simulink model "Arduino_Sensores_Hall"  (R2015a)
settings: Solver=ode45  StartTime=0.0  StopTime=10.0  RelTol=1e-3
libraries: arduinolib x10, dspsigops x9, simulink x7

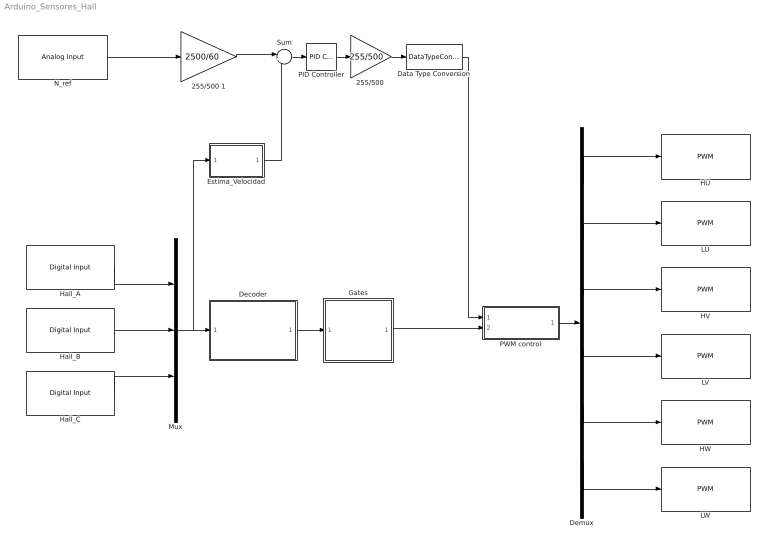
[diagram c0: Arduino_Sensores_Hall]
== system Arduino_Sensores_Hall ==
  "255/500 " : Gain  Gain=255/500
  255/500 1 : Gain  Gain=2500/60
  Data Type Conversion : DataTypeConversion  OutDataTypeStr=int16  RndMeth=Round
  Decoder : Subsystem
  Demux : Demux  Outputs=6
  Estima_Velocidad : Subsystem
  Gates : Subsystem
  HU : arduinolib/PWM  pinNumber=3  blockPlatform=arduino
  HV : arduinolib/PWM  pinNumber=6  blockPlatform=arduino
  HW : arduinolib/PWM  pinNumber=10  blockPlatform=arduino
  Hall_A : arduinolib/Digital Input  pinNumber=8  sampleTime=1  blockPlatform=arduino
  Hall_B : arduinolib/Digital Input  pinNumber=12  sampleTime=1  blockPlatform=arduino
  Hall_C : arduinolib/Digital Input  pinNumber=13  sampleTime=1  blockPlatform=arduino
  LU : arduinolib/PWM  pinNumber=5  blockPlatform=arduino
  LV : arduinolib/PWM  pinNumber=9  blockPlatform=arduino
  LW : arduinolib/PWM  pinNumber=11  blockPlatform=arduino
  Mux : Mux  Inputs=3
  N_ref : arduinolib/Analog Input  pinNumber=0  sampleTime=1  blockPlatform=arduino
  PID Controller : simulink/Continuous/PID Controller  Controller=PID  TimeDomain=Continuous-time  SampleTime=-1  IntegratorMethod=Forward Euler  FilterMethod=Forward Euler  Form=Parallel  UseFilter=on  ControllerParametersSource=internal  P=500  I=0.1  D=0.08  N=1  InitialConditionSource=internal  InitialConditionForIntegrator=0  InitialConditionForFilter=0  ExternalReset=none  LimitOutput=off  UpperSaturationLimit=inf  LowerSaturationLimit=-inf  LinearizeAsGain=on  AntiWindupMode=none  Kb=1  TrackingMode=off  Kt=1  PParamMin=[]  PParamMax=[]  IParamMin=[]  IParamMax=[]  DParamMin=[]  DParamMax=[]  NParamMin=[]  NParamMax=[]  KbParamMin=[]  KbParamMax=[]  KtParamMin=[]  KtParamMax=[]  POutMin=[]  POutMax=[]  IOutMin=[]  IOutMax=[]  DOutMin=[]  DOutMax=[]  NOutMin=[]  NOutMax=[]  KbOutMin=[]  KbOutMax=[]  KtOutMin=[]  KtOutMax=[]  IntegratorOutMin=[]  IntegratorOutMax=[]  FilterOutMin=[]  FilterOutMax=[]  SumOutMin=[]  SumOutMax=[]  SumI1OutMin=[]  SumI1OutMax=[]  SumI2OutMin=[]  SumI2OutMax=[]  SumI3OutMin=[]  SumI3OutMax=[]  SumDOutMin=[]  SumDOutMax=[]  SaturationOutMin=[]  SaturationOutMax=[]  IntegratorContinuousStateAttributes=''  IntegratorStateMustResolveToSignalObject=off  IntegratorRTWStateStorageClass=Auto  FilterContinuousStateAttributes=''  FilterStateMustResolveToSignalObject=off  FilterRTWStateStorageClass=Auto  DifferentiatorICPrevScaledInput=0  DifferentiatorOutMin=[]  DifferentiatorOutMax=[]
  PWM control : Subsystem
  Sum : Sum  Inputs=|+-
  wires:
  Hall_B/1 -> Mux/2
  Hall_A/1 -> Mux/1
  Hall_C/1 -> Mux/3
  Mux/1 -> Estima_Velocidad/1(Hall), Decoder/1("Hall ")
  Gates/1(Gates) -> PWM control/2(Gates)
  Sum/1 -> PID Controller/1
  PID Controller/1 -> "255/500 "/1
  Decoder/1(emf_abc) -> Gates/1("emf_abc ")
  "255/500 "/1 -> Data Type Conversion/1
  Data Type Conversion/1 -> PWM control/1(V control)
  PWM control/1(Pulsos) -> Demux/1
  Demux/1 -> HU/1
  Demux/2 -> LU/1
  Demux/3 -> HV/1
  Demux/4 -> LV/1
  Demux/5 -> HW/1
  Demux/6 -> LW/1
  Estima_Velocidad/1(N_est) -> Sum/2
  255/500 1/1 -> Sum/1
  N_ref/1 -> 255/500 1/1

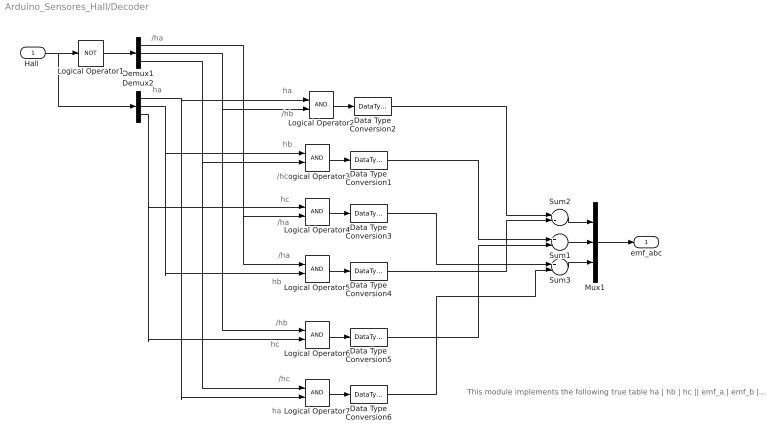
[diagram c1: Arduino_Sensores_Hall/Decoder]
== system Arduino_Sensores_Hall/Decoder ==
  note: /ha
  note: ha
  note: ha
  note: /hb
  note: hb
  note: /hc
  note: hc
  note: /ha
  note: /ha
  note: hb
  note: /hb
  note: hc
  note: /hc
  note: ha
  note: This module implements the following true table ha | hb | hc || emf_a | emf_b | emf_c -------------------------------------------------------------------------------- 0 0 0 0 0 0 0 0 1 0 -1 +1 0 1 0 -1 +1 0 0 1 1 -1 0 +1 1 0 0 +1 0 -1 1 0 1 +1 -1 0 1 1 0 0 +1 -1 1 1 1 0 0 0
  "Hall " : Inport
  Data Type Conversion{1..6} (6 alike) : DataTypeConversion
  Demux1 : Demux  Outputs=3
  Demux2 : Demux  Outputs=3
  Logical Operator1 : Logic  Operator=NOT  AllPortsSameDT=off  OutDataTypeStr=boolean
  Logical Operator{2..7} (6 alike) : Logic  AllPortsSameDT=off  OutDataTypeStr=boolean
  Mux1 : Mux  Inputs=3
  Sum1 : Sum  Inputs=+-  OutDataTypeStr=double
  Sum2 : Sum  Inputs=+-  OutDataTypeStr=double
  Sum3 : Sum  Inputs=+-  OutDataTypeStr=double
  emf_abc : Outport
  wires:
  "Hall "/1 -> Logical Operator1/1, Demux2/1
  Logical Operator1/1 -> Demux1/1
  Demux2/3 -> Logical Operator4/1, Logical Operator6/2
  Demux2/2 -> Logical Operator3/1, Logical Operator5/2
  Demux2/1 -> Logical Operator2/1, Logical Operator7/2
  Demux1/3 -> Logical Operator3/2, Logical Operator7/1
  Demux1/2 -> Logical Operator2/2, Logical Operator6/1
  Demux1/1 -> Logical Operator4/2, Logical Operator5/1
  Logical Operator2/1 -> Data Type Conversion2/1
  Sum2/1 -> Mux1/1
  Sum1/1 -> Mux1/2
  Sum3/1 -> Mux1/3
  Mux1/1 -> emf_abc/1
  Logical Operator3/1 -> Data Type Conversion1/1
  Logical Operator4/1 -> Data Type Conversion3/1
  Logical Operator5/1 -> Data Type Conversion4/1
  Logical Operator6/1 -> Data Type Conversion5/1
  Logical Operator7/1 -> Data Type Conversion6/1
  Data Type Conversion2/1 -> Sum2/1
  Data Type Conversion4/1 -> Sum2/2
  Data Type Conversion1/1 -> Sum1/1
  Data Type Conversion5/1 -> Sum1/2
  Data Type Conversion3/1 -> Sum3/1
  Data Type Conversion6/1 -> Sum3/2

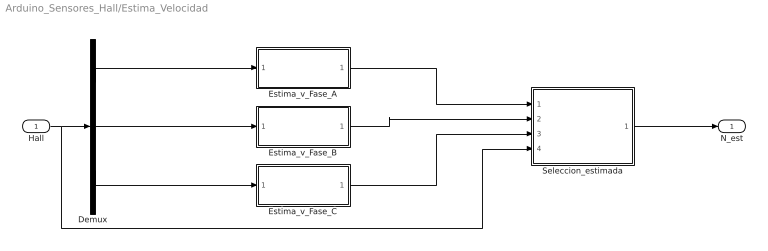
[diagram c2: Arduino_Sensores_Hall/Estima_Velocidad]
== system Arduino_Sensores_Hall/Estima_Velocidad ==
  Hall : Inport
  Demux : Demux  Outputs=3
  Estima_v_Fase_A : Subsystem
  Estima_v_Fase_B : Subsystem
  Estima_v_Fase_C : Subsystem
  Seleccion_estimada : Subsystem
  N_est : Outport
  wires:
  Demux/1 -> Estima_v_Fase_A/1(Hall_i)
  Hall/1 -> Seleccion_estimada/4(Hall), Demux/1
  Demux/3 -> Estima_v_Fase_C/1(Hall_i)
  Demux/2 -> Estima_v_Fase_B/1(Hall_i)
  Estima_v_Fase_A/1(Estimada_i) -> Seleccion_estimada/1(Estimada_A)
  Estima_v_Fase_B/1(Estimada_i) -> Seleccion_estimada/2(Estimada_B)
  Estima_v_Fase_C/1(Estimada_i) -> Seleccion_estimada/3(Estimada_C)
  Seleccion_estimada/1(Out1) -> N_est/1

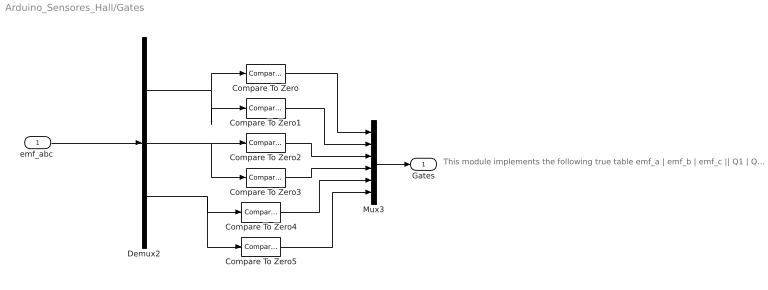
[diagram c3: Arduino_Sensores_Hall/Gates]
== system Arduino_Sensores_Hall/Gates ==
  note: This module implements the following true table emf_a | emf_b | emf_c || Q1 | Q2 | Q3 | Q4 | Q5 | Q6 ------------------------------------------------------------------------------------------------------------------ 0 0 0 0 0 0 0 0 0 0 -1 +1 0 0 0 1 1 0 -1 +1 0 0 1 1 0 0 0 -1 0 +1 0 1 0 0 1 0 +1 0 -1 1 0 0 0 0 1 +1 -1 0 1 0 0 1 0 0 0 +1 -1 0 0 1 0 0 1 0 0 0 0 0 0 0 0 0
  "emf_abc " : Inport
  Compare To Zero : simulink/Logic and Bit Operations/Compare To Zero  relop=>  OutDataTypeStr=boolean  ZeroCross=off
  Compare To Zero1 : simulink/Logic and Bit Operations/Compare To Zero  relop=<  OutDataTypeStr=boolean  ZeroCross=off
  Compare To Zero2 : simulink/Logic and Bit Operations/Compare To Zero  relop=>  OutDataTypeStr=boolean  ZeroCross=off
  Compare To Zero3 : simulink/Logic and Bit Operations/Compare To Zero  relop=<  OutDataTypeStr=boolean  ZeroCross=off
  Compare To Zero4 : simulink/Logic and Bit Operations/Compare To Zero  relop=>  OutDataTypeStr=boolean  ZeroCross=off
  Compare To Zero5 : simulink/Logic and Bit Operations/Compare To Zero  relop=<  OutDataTypeStr=boolean  ZeroCross=off
  Demux2 : Demux  Outputs=3
  Mux3 : Mux  Inputs=6
  Gates : Outport
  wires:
  "emf_abc "/1 -> Demux2/1
  Mux3/1 -> Gates/1
  Demux2/1 -> Compare To Zero/1, Compare To Zero1/1
  Demux2/2 -> Compare To Zero2/1, Compare To Zero3/1
  Demux2/3 -> Compare To Zero4/1, Compare To Zero5/1
  Compare To Zero/1 -> Mux3/1
  Compare To Zero1/1 -> Mux3/2
  Compare To Zero2/1 -> Mux3/3
  Compare To Zero3/1 -> Mux3/4
  Compare To Zero4/1 -> Mux3/5
  Compare To Zero5/1 -> Mux3/6

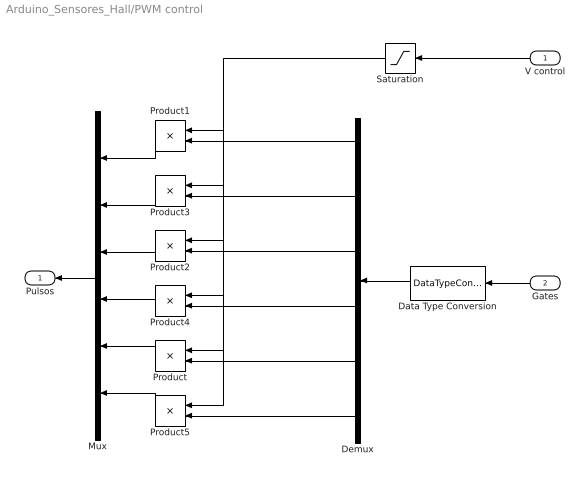
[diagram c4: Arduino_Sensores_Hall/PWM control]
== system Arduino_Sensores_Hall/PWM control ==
  V control : Inport
  Gates : Inport  Port=2
  Data Type Conversion : DataTypeConversion  OutDataTypeStr=double
  Demux : Demux  Outputs=6
  Mux : Mux  Inputs=6
  Product{,1..5} (6 alike) : Product
  Saturation : Saturate  UpperLimit=255  LowerLimit=0
  Pulsos : Outport
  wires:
  Gates/1 -> Data Type Conversion/1
  Data Type Conversion/1 -> Demux/1
  Mux/1 -> Pulsos/1
  Product1/1 -> Mux/1
  Product2/1 -> Mux/3
  Product/1 -> Mux/5
  Demux/5 -> Product/2
  Demux/3 -> Product2/2
  Demux/1 -> Product1/2
  V control/1 -> Saturation/1
  Product5/1 -> Mux/6
  Demux/6 -> Product5/2
  Product4/1 -> Mux/4
  Demux/4 -> Product4/2
  Product3/1 -> Mux/2
  Demux/2 -> Product3/2
  Saturation/1 -> Product3/1, Product4/1, Product/1, Product5/1, Product2/1, Product1/1

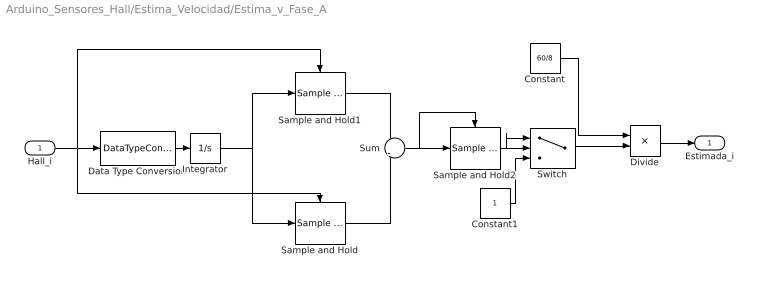
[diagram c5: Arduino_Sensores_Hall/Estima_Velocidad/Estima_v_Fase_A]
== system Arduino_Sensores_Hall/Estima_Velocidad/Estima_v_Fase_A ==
  Hall_i : Inport
  Constant : Constant  Value=60/8
  Constant1 : Constant
  Data Type Conversion : DataTypeConversion  OutDataTypeStr=double
  Divide : Product  Inputs=*/
  Integrator : Integrator
  Sample and Hold : dspsigops/Sample and Hold  trig=Rising edge  initCond=0  latchinput=off
  Sample and Hold1 : dspsigops/Sample and Hold  trig=Falling edge  initCond=0  latchinput=off
  Sample and Hold2 : dspsigops/Sample and Hold  trig=Rising edge  initCond=0  latchinput=off
  Sum : Sum  Inputs=+|-
  Switch : Switch  Criteria=u2 > Threshold
  Estimada_i : Outport
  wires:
  Hall_i/1 -> Data Type Conversion/1, Sample and Hold/Trigger, Sample and Hold1/Trigger
  Integrator/1 -> Sample and Hold1/1, Sample and Hold/1
  Sample and Hold/1 -> Sum/2
  Sample and Hold1/1 -> Sum/1
  Sum/1 -> Sample and Hold2/Trigger, Sample and Hold2/1
  Sample and Hold2/1 -> Switch/1, Switch/2
  Constant/1 -> Divide/1
  Switch/1 -> Divide/2
  Constant1/1 -> Switch/3
  Divide/1 -> Estimada_i/1
  Data Type Conversion/1 -> Integrator/1

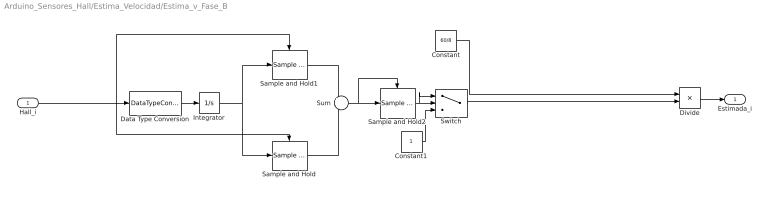
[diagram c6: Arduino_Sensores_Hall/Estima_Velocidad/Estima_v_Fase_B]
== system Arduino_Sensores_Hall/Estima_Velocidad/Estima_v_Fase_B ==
  Hall_i : Inport
  Constant : Constant  Value=60/8
  Constant1 : Constant
  Data Type Conversion : DataTypeConversion  OutDataTypeStr=double
  Divide : Product  Inputs=*/
  Integrator : Integrator
  Sample and Hold : dspsigops/Sample and Hold  trig=Rising edge  initCond=0  latchinput=off
  Sample and Hold1 : dspsigops/Sample and Hold  trig=Falling edge  initCond=0  latchinput=off
  Sample and Hold2 : dspsigops/Sample and Hold  trig=Rising edge  initCond=0  latchinput=off
  Sum : Sum  Inputs=+|-
  Switch : Switch  Criteria=u2 > Threshold
  Estimada_i : Outport
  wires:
  Hall_i/1 -> Sample and Hold/Trigger, Sample and Hold1/Trigger, Data Type Conversion/1
  Integrator/1 -> Sample and Hold1/1, Sample and Hold/1
  Sample and Hold/1 -> Sum/2
  Sample and Hold1/1 -> Sum/1
  Sum/1 -> Sample and Hold2/Trigger, Sample and Hold2/1
  Sample and Hold2/1 -> Switch/1, Switch/2
  Constant/1 -> Divide/1
  Switch/1 -> Divide/2
  Constant1/1 -> Switch/3
  Divide/1 -> Estimada_i/1
  Data Type Conversion/1 -> Integrator/1

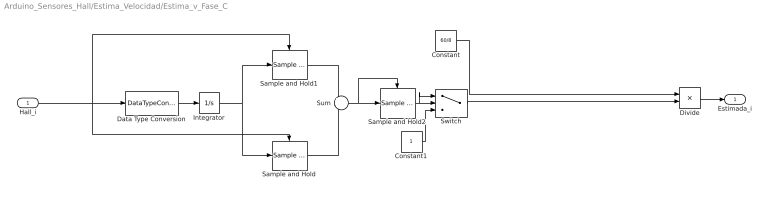
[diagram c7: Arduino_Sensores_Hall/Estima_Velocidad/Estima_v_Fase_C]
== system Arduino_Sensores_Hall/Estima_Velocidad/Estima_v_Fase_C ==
  Hall_i : Inport
  Constant : Constant  Value=60/8
  Constant1 : Constant
  Data Type Conversion : DataTypeConversion  OutDataTypeStr=double
  Divide : Product  Inputs=*/
  Integrator : Integrator
  Sample and Hold : dspsigops/Sample and Hold  trig=Rising edge  initCond=0  latchinput=off
  Sample and Hold1 : dspsigops/Sample and Hold  trig=Falling edge  initCond=0  latchinput=off
  Sample and Hold2 : dspsigops/Sample and Hold  trig=Rising edge  initCond=0  latchinput=off
  Sum : Sum  Inputs=+|-
  Switch : Switch  Criteria=u2 > Threshold  Threshold=3E-5
  Estimada_i : Outport
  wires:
  Hall_i/1 -> Data Type Conversion/1, Sample and Hold/Trigger, Sample and Hold1/Trigger
  Integrator/1 -> Sample and Hold1/1, Sample and Hold/1
  Sample and Hold/1 -> Sum/2
  Sample and Hold1/1 -> Sum/1
  Sum/1 -> Sample and Hold2/Trigger, Sample and Hold2/1
  Sample and Hold2/1 -> Switch/1, Switch/2
  Constant/1 -> Divide/1
  Switch/1 -> Divide/2
  Constant1/1 -> Switch/3
  Divide/1 -> Estimada_i/1
  Data Type Conversion/1 -> Integrator/1

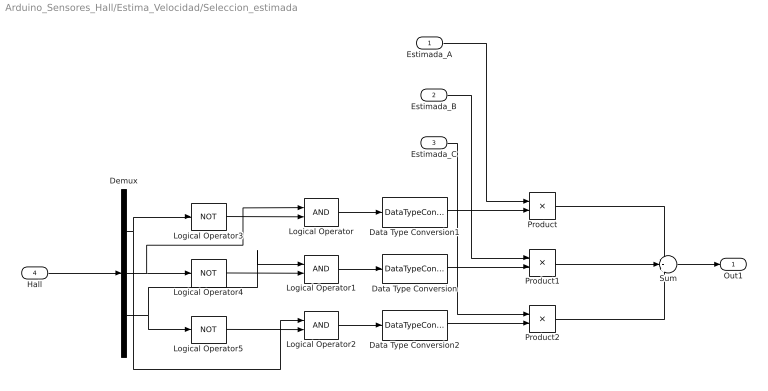
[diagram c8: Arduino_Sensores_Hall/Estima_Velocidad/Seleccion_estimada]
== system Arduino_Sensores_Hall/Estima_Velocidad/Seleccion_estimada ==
  Estimada_A : Inport
  Estimada_B : Inport  Port=2
  Estimada_C : Inport  Port=3
  Hall : Inport  Port=4
  Data Type Conversion : DataTypeConversion  OutDataTypeStr=double
  Data Type Conversion1 : DataTypeConversion  OutDataTypeStr=double
  Data Type Conversion2 : DataTypeConversion  OutDataTypeStr=double
  Demux : Demux  Outputs=3
  Logical Operator : Logic  IconShape=distinctive  AllPortsSameDT=off  OutDataTypeStr=boolean
  Logical Operator1 : Logic  IconShape=distinctive  AllPortsSameDT=off  OutDataTypeStr=boolean
  Logical Operator2 : Logic  IconShape=distinctive  AllPortsSameDT=off  OutDataTypeStr=boolean
  Logical Operator3 : Logic  Operator=NOT  IconShape=distinctive  AllPortsSameDT=off  OutDataTypeStr=boolean
  Logical Operator4 : Logic  Operator=NOT  IconShape=distinctive  AllPortsSameDT=off  OutDataTypeStr=boolean
  Logical Operator5 : Logic  Operator=NOT  IconShape=distinctive  AllPortsSameDT=off  OutDataTypeStr=boolean
  Product : Product
  Product1 : Product
  Product2 : Product
  Sum : Sum  Inputs=+++
  Out1 : Outport
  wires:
  Hall/1 -> Demux/1
  Product/1 -> Sum/1
  Product1/1 -> Sum/2
  Product2/1 -> Sum/3
  Logical Operator3/1 -> Logical Operator/2
  Logical Operator4/1 -> Logical Operator1/2
  Logical Operator5/1 -> Logical Operator2/2
  Demux/3 -> Logical Operator1/1, Logical Operator5/1
  Demux/2 -> Logical Operator/1, Logical Operator4/1
  Demux/1 -> Logical Operator2/1, Logical Operator3/1
  Logical Operator1/1 -> Data Type Conversion/1
  Logical Operator2/1 -> Data Type Conversion2/1
  Logical Operator/1 -> Data Type Conversion1/1
  Sum/1 -> Out1/1
  Estimada_C/1 -> Product2/1
  Data Type Conversion2/1 -> Product2/2
  Data Type Conversion/1 -> Product1/2
  Data Type Conversion1/1 -> Product/2
  Estimada_B/1 -> Product1/1
  Estimada_A/1 -> Product/1
